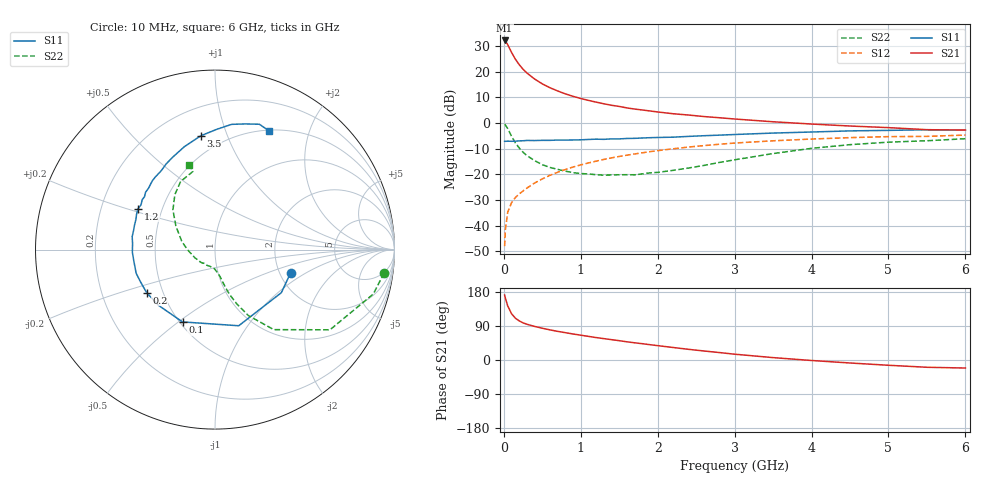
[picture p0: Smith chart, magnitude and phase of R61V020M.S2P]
! SIEMENS Small Signal Semiconductors
! BFR193
! Si NPN RF Bipolar Junction Transistor in SOT23
! VCE = 1 V  IC = 20 mA
! Common Emitter S-Parameters:  May  1996
# GHz  S  MA  R  50
!  f  S11  S21  S12  S22
! GHz  MAG  ANG  MAG  ANG  MAG  ANG  MAG  ANG
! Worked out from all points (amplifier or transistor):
!   36 points, 10 MHz to 6 GHz, reference 50 ohm
!   highest |S21| = 32.2 dB at 10 MHz (marker M1)
!   |S21| within 3 dB of that: start of sweep to 72.81 MHz
!   unconditionally stable (mu >= 1): 498.4 MHz to 2.229 GHz
!   at 250 MHz: K = 0.85, MSG = 23.7 dB, |S12| = -26.4 dB
!   at 1.4 GHz: K = 1.03, MAG = 9.2 dB, |S12| = -13.6 dB
!   at 6 GHz: K = 0.97, MSG = 1.0 dB, |S12| = -4.7 dB
!   S11 on the Smith chart (normalised r, x): 10 MHz: 2.30, -0.73; 100 MHz: 0.52, -0.52; 200 MHz: 0.41, -0.24; 1.2 GHz: 0.36, +0.22; 3.5 GHz: 0.38, +0.81; 6 GHz: 0.51, +1.43
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0.01  0.4412 -16.9  40.66 171.6  0.004 84.9  0.9512 -7.9
0.02  0.4407 -33.0  39.59 163.3  0.0083 79.4  0.9158 -15.7
0.05  0.4444 -72.7  33.73 143.0  0.0183 67.5  0.781 -34.9
0.1  0.4417 -114.2  23.83 122.1  0.0281 60.5  0.5534 -53.7
0.15  0.4423 -135.5  17.55 110.4  0.0355 59.5  0.4113 -63.2
0.2  0.4501 -147.9  13.74 103.2  0.0416 60.7  0.3276 -68.0
0.25  0.4524 -156.7  11.2 98.0  0.0476 62.1  0.2698 -71.5
0.3  0.4586 -163.3  9.444 94.3  0.0542 64.0  0.2324 -73.7
0.4  0.4569 -172.5  7.209 88.6  0.068 65.9  0.1854 -76.7
0.5  0.4607 -178.2  5.8 83.8  0.0817 66.7  0.1545 -79.2
0.6  0.4605 175.7  4.875 79.5  0.096 66.9  0.1367 -82.0
0.7  0.4671 171.1  4.219 75.5  0.1102 66.9  0.1253 -84.8
0.8  0.466 166.7  3.704 72.1  0.1246 66.4  0.1158 -88.1
0.9  0.4687 163.2  3.318 68.6  0.139 65.6  0.1081 -90.6
1.1  0.4795 155.7  2.766 62.3  0.1673 63.7  0.1019 -98.9
1.2  0.4858 152.0  2.557 59.2  0.1813 62.6  0.0988 -103.8
1.6  0.5017 140.4  1.974 48.0  0.2369 57.2  0.0986 -124.5
2.2  0.5313 124.5  1.52 33.0  0.3157 48.4  0.1199 -156.8
3.5  0.6387 97.2  1.06 6.3  0.4515 27.6  0.2547 148.9
4.5  0.7041 82.4  0.876 -7.9  0.5207 13.4  0.3796 126.1
5.5  0.7409 70.5  0.743 -19.2  0.5504 -0.3  0.4524 105.8
6  0.7267 65.5  0.731 -21.2  0.5841 -4.4  0.4955 107.0
